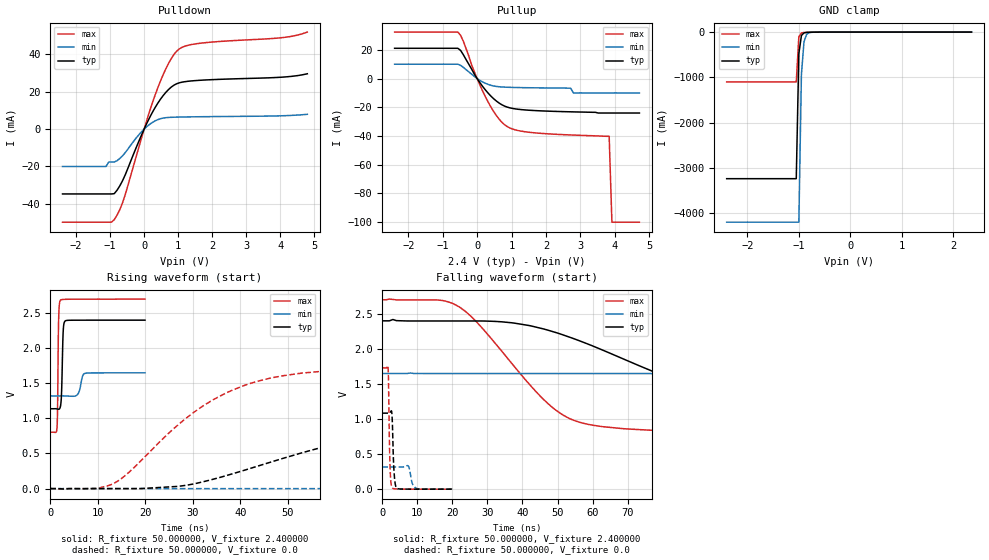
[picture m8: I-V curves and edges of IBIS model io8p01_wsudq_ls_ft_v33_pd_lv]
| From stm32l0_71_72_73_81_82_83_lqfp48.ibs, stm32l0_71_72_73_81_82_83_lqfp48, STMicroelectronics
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|   Model io8p01_wsudq_ls_ft_v33_pd_lv
[Model]  io8p01_wsudq_ls_ft_v33_pd_lv
Model_type I/O
Polarity   Non-Inverting
Enable   Active-Low
Vinl =   0.720000V
Vinh =   1.680000V
Vmeas =  1.200000V
Cref =   50.000000pF
Rref =   100.000000M
Vref =   0.0V
C_comp   2.582000pF   2.574200pF   2.601000pF
[Temperature Range]   25.000000   0.105000k   -40.000000
[Pullup Reference]   2.400000V   1.650000V   2.700000V
[Pulldown Reference]   0.0V   0.0V   0.0V
[POWER Clamp Reference]   2.400000V   1.650000V   2.700000V
[GND Clamp Reference]   0.0V   0.0V   0.0V
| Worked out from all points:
|   slope of the pulldown table from 0 to 0.36 V, typ, clamps not added: 28.5 ohm
|   slope of the pullup table from 0 to 0.36 V, typ, clamps not added: 32.2 ohm
|   GND clamp passes 1 mA (typ) near -0.64 V on its own axis
|   rising waveform, R_fixture 50.000000, V_fixture 2.400000: 20-80 % time 278ps typ, 628ps min, 193ps max; typ from 1.14 V to 2.4 V
|   rising waveform, R_fixture 50.000000, V_fixture 0.0: 20-80 % time 39.7ns typ, 106ns min, 19.4ns max; typ from 0 V to 1.08 V
|   falling waveform, R_fixture 50.000000, V_fixture 2.400000: 20-80 % time 40.9ns typ, 106ns min, 20.1ns max; typ from 2.4 V to 1.14 V
|   falling waveform, R_fixture 50.000000, V_fixture 0.0: 20-80 % time 475ps typ, 848ps min, 374ps max; typ from 1.08 V to 0 V
[Pulldown]
|Voltage   I(typ)   I(min)   I(max)
-2.4V     -34.7mA    -20mA      -49.82mA
-1.12V    -34.7mA    -20mA      -49.82mA
-1.04V    -34.7mA    -17.6mA    -49.82mA
-880mV    -34.55mA   -17.6mA    -48.46mA
-560mV    -24.65mA   -12.68mA   -35.33mA
0V        0A         0A         142fA
400mV     13.84mA    5.066mA    22.03mA
720mV     21.25mA    6.254mA    35.26mA
1.04V     24.83mA    6.464mA    43.03mA
1.6V      26.11mA    6.627mA    45.88mA
4V        27.76mA    7.125mA    48.88mA
4.8V      29.64mA    7.94mA     51.96mA
[Pullup]
|Voltage   I(typ)   I(min)   I(max)
-2.4V     21.06mA    9.987mA    32.34mA
-560mV    21.06mA    9.987mA    32.34mA
-400mV    16.53mA    7.734mA    25.89mA
-80mV     3.011mA    1.498mA    4.671mA
320mV     -10.16mA   -4.078mA   -16.34mA
640mV     -17.08mA   -5.718mA   -28.28mA
960mV     -20.45mA   -6.129mA   -34.5mA
1.76V     -22.39mA   -6.471mA   -37.97mA
2.8V      -23.2mA    -10mA      -39.35mA
3.84V     -24mA      -10mA      -40.2mA
3.92V     -24mA      -10mA      -100mA
4.72V     -24mA      -10mA      -100mA
[GND_clamp]
|Voltage   I(typ)   I(min)   I(max)
-2.4V     -3.237A    -4.198A    -1.1A
-1.05V    -3.237A    -4.198A    -1.1A
-1V       -475.9mA   -4.198A    -104.3mA
-950mV    -76.38mA   -935.5mA   -18.57mA
-900mV    -16.78mA   -213mA     -9.302mA
-850mV    -6.726mA   -51.1mA    -6.732mA
-800mV    -4.12mA    -13.96mA   -4.933mA
-650mV    -1.06mA    -1.216mA   -1.157mA
2.35V     52.69uA    50.02uA    36.84uA
[POWER_clamp]
|Voltage   I(typ)   I(min)   I(max)
-2.4V     0A         0A         0A
0V        0A         0A         0A
[Ramp]
| variable   typ   min   max
dV/dt_r  0.65004/39.65230n   0.18952/0.10644u   1.03746/19.32561n
dV/dt_f  0.75702/40.82500n   0.19512/0.10569u   1.13800/20.05288n
R_load = 50.000000
[Rising Waveform]
R_fixture= 50.000000
V_fixture= 2.400000
V_fixture_min= 1.650000
V_fixture_max= 2.700000
|time   V(typ)   V(min)   V(max)
0s        1.137V     1.32V      802.8mV
1.401ns   1.135V     1.32V      852mV
1.522ns   1.133V     1.32V      1.088V
1.762ns   1.13V      1.32V      2.412V
2.122ns   1.166V     1.32V      2.682V
2.362ns   1.344V     1.32V      2.691V
2.723ns   2.245V     1.32V      2.694V
3.083ns   2.383V     1.32V      2.695V
7.247ns   2.399V     1.639V     2.698V
19.94ns   2.399V     1.649V     2.7V
[Rising Waveform]
R_fixture= 50.000000
V_fixture= 0.0
V_fixture_min= 0.0
V_fixture_max= 0.0
|time   V(typ)   V(min)   V(max)
0s        1.421nV    7.15nV     1.172nV
13.01ns   -217.8uV   -47.5uV    61.14mV
29.03ns   52.01mV    -46.28uV   1.025V
38.04ns   204.7mV    -46.19uV   1.393V
47.05ns   390.4mV    -34.44uV   1.583V
60.06ns   636.1mV    18.97uV    1.686V
84.08ns   914.9mV    996.4uV    1.724V
120.1ns   1.052V     36.65mV    1.729V
253.3ns   1.083V     266.3mV    1.729V
498.5ns   1.083V     316.1mV    1.729V
[Falling Waveform]
R_fixture= 50.000000
V_fixture= 2.400000
V_fixture_min= 1.650000
V_fixture_max= 2.700000
|time   V(typ)   V(min)   V(max)
0s        2.399V     1.649V     2.7V
21.02ns   2.397V     1.648V     2.623V
37.04ns   2.371V     1.648V     1.786V
50.05ns   2.225V     1.648V     1.108V
57.06ns   2.1V       1.648V     943.3mV
69.07ns   1.85V      1.648V     860.8mV
99.1ns    1.353V     1.647V     814.4mV
145.1ns   1.183V     1.626V     804mV
287.3ns   1.138V     1.379V     802.8mV
498.5ns   1.137V     1.32V      802.8mV
[Falling Waveform]
R_fixture= 50.000000
V_fixture= 0.0
V_fixture_min= 0.0
V_fixture_max= 0.0
|time   V(typ)   V(min)   V(max)
0s        1.083V     316.1mV    1.729V
1.642ns   1.083V     316.1mV    1.73V
2.162ns   1.086V     316.1mV    372.3mV
2.402ns   1.105V     316.1mV    114mV
2.763ns   1.045V     316.1mV    23.77mV
3.283ns   290.2mV    316.1mV    6.194mV
4.004ns   19.5mV     316.1mV    3.345mV
7.367ns   651.1uV    332.3mV    83.84uV
9.65ns    143.2uV    13.78mV    -25.72uV
19.94ns   1.421nV    7.15nV     1.172nV
